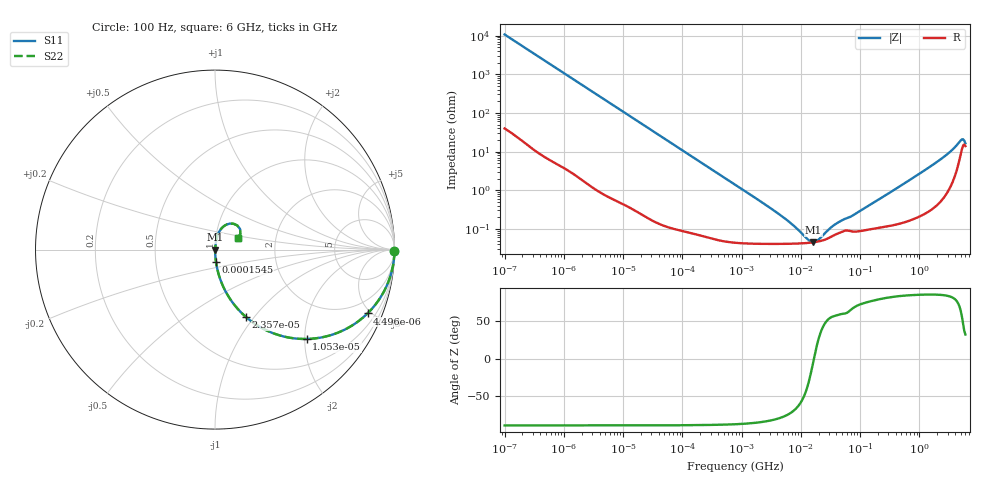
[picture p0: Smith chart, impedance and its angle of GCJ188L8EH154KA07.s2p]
!Murata Part Number: GCJ188L8EH154KA07
!These Parameters are Measured in Series Mode Connection
!Data Generated on Mar 13, 2026
!  o--ll--o
!Port1  Port2
!  o------o
!Operation Temp=25[degC], DC Bias Voltage=0[V]
!Freq. Start=100[Hz] Stop=6[GHz] 401[Steps]
# Hz S RI R 50
!Freq.(Hz) S11(Real) S11(Imag) S21(Real) S21(Imag) S12(Real) S12(Imag) S22(Real) S22(Imag)
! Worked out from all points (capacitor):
!   401 points, 100 Hz to 6 GHz, reference 50 ohm
!   read as one part in series: C = 149 nF near 109 Hz
!   lowest |Z| = 45 mohm at 16.27 MHz (marker M1)
!   series resonance near 16.68 MHz, so ESL is about 610 pH
!   S11 on the Smith chart (normalised r, x): 100 Hz: open; 4.496 kHz: 1.02, -4.77; 10.53 kHz: 1.01, -2.04; 23.57 kHz: 1.00, -0.91; 154.5 kHz: 1.00, -0.14; 6 GHz: 1.28, +0.17
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100  0.9999 -0.00939  0.000123 0.00939  0.000123 0.00939  0.9999 -0.00939
600  0.9967 -0.0559  0.00332 0.0559  0.00332 0.0559  0.9967 -0.0559
2008  0.9655 -0.1808  0.0345 0.1808  0.0345 0.1808  0.9655 -0.1808
4496  0.8499 -0.3555  0.1501 0.3555  0.1501 0.3555  0.8499 -0.3555
10527  0.5105 -0.4979  0.4895 0.4979  0.4895 0.4979  0.5105 -0.4979
23569  0.174 -0.3768  0.826 0.3768  0.826 0.3768  0.174 -0.3768
40335  0.0678 -0.2489  0.9322 0.2489  0.9322 0.2489  0.0678 -0.2489
154540  0.00562 -0.0696  0.9944 0.0696  0.9944 0.0696  0.00562 -0.0696
774597  0.000634 -0.014  0.9994 0.014  0.9994 0.014  0.000634 -0.014
4856642  0.000414 -0.00205  0.9996 0.00205  0.9996 0.00205  0.000414 -0.00205
1.300572e7  0.000433 -0.000328  0.9996 0.000328  0.9996 0.000328  0.000433 -0.000328
1.555665e7  0.000445 -9.08e-05  0.9996 9.08e-05  0.9996 9.08e-05  0.000445 -9.08e-05
1.626902e7  0.000449 -3.24e-05  0.9996 3.24e-05  0.9996 3.24e-05  0.000449 -3.24e-05
1.946e7  0.00047 0.000201  0.9995 -0.000201  0.9995 -0.000201  0.00047 0.000201
3.983537e7  0.000733 0.00116  0.9993 -0.00116  0.9993 -0.00116  0.000733 0.00116
7.455971e7  0.00086 0.00203  0.9991 -0.00203  0.9991 -0.00203  0.00086 0.00203
3.124326e8  0.00126 0.00842  0.9987 -0.00842  0.9987 -0.00842  0.00126 0.00842
2.142435e9  0.00789 0.0576  0.9921 -0.0576  0.9921 -0.0576  0.00789 0.0576
3.666503e9  0.0281 0.1074  0.9719 -0.1074  0.9719 -0.1074  0.0281 0.1074
4.796499e9  0.0829 0.1448  0.9171 -0.1448  0.9171 -0.1448  0.0829 0.1448
5.245841e9  0.124 0.1348  0.876 -0.1348  0.876 -0.1348  0.124 0.1348
6e9  0.1265 0.0668  0.8735 -0.0668  0.8735 -0.0668  0.1265 0.0668
